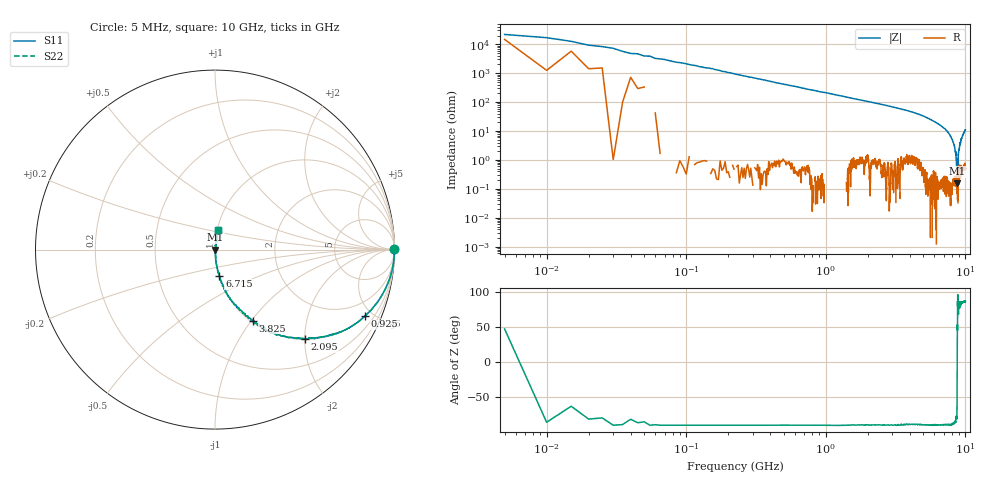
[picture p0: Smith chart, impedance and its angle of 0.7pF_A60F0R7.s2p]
! Amotech Co.,Ltd.
! http://www.amotech.co.kr/
! Part Number: A60F0R7
! These Parameters are Measured in Series Mode Connection
! Operation Temp=25[degC], DC Bias Voltage=0[V]
! Freq. Start=5[MHz] Stop=10[GHz], 2000[Steps]
! Date: Monday, July 20, 2020, 03:12:17
# GHZ S RI R 50.000000
!Freq.(Hz) S11(Real) S11(Imag) S21(Real) S21(Imag) S12(Real) S12(Imag) S22(Real) S22(Imag)
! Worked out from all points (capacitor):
!   2000 points, 5 MHz to 10 GHz, reference 50 ohm
!   read as one part in series: C = 763 fF near 55 MHz
!   lowest |Z| = 158 mohm at 8.72 GHz (marker M1)
!   series resonance near 8.732 GHz, so ESL is about 440 pH
!   S11 on the Smith chart (normalised r, x): 5 MHz: open; 925 MHz: 1.00, -4.51; 2.095 GHz: 1.01, -2.01; 3.825 GHz: 1.02, -1.02; 6.715 GHz: 1.00, -0.30; 10 GHz: 1.01, +0.22
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0.005  0.9969 0.00336  0.00309 -0.00336  0.00309 -0.00336  0.9969 0.00336
0.09  0.9981 -0.0431  0.00188 0.0431  0.00188 0.0431  0.9981 -0.0431
0.24  0.9871 -0.1127  0.0129 0.1127  0.0129 0.1127  0.9871 -0.1127
0.49  0.9464 -0.2241  0.0536 0.2241  0.0536 0.2241  0.9464 -0.2241
0.925  0.8355 -0.3706  0.1645 0.3706  0.1645 0.3706  0.8355 -0.3706
1.675  0.6107 -0.4846  0.3893 0.4846  0.3893 0.4846  0.6107 -0.4846
2.095  0.502 -0.497  0.498 0.497  0.498 0.497  0.502 -0.497
3.34  0.2652 -0.4395  0.7348 0.4395  0.7348 0.4395  0.2652 -0.4395
3.825  0.2106 -0.3959  0.7894 0.3959  0.7894 0.3959  0.2106 -0.3959
5.005  0.0985 -0.2934  0.9015 0.2934  0.9015 0.2934  0.0985 -0.2934
6.67  0.0246 -0.1502  0.9754 0.1502  0.9754 0.1502  0.0246 -0.1502
6.715  0.0241 -0.1466  0.9759 0.1466  0.9759 0.1466  0.0241 -0.1466
7.7  0.00689 -0.0771  0.9931 0.0771  0.9931 0.0771  0.00689 -0.0771
8.335  0.00288 -0.0305  0.9971 0.0305  0.9971 0.0305  0.00288 -0.0305
8.545  0.00242 -0.0148  0.9976 0.0148  0.9976 0.0148  0.00242 -0.0148
8.72  0.00128 -0.000914  0.9987 0.000914  0.9987 0.000914  0.00128 -0.000914
8.755  0.00418 0.00265  0.9958 -0.00265  0.9958 -0.00265  0.00418 0.00265
8.815  -0.000866 0.00785  1.001 -0.00785  1.001 -0.00785  -0.000866 0.00785
8.935  0.0066 0.0179  0.9934 -0.0179  0.9934 -0.0179  0.0066 0.0179
9.135  0.00698 0.034  0.993 -0.034  0.993 -0.034  0.00698 0.034
9.515  0.01 0.0656  0.99 -0.0656  0.99 -0.0656  0.01 0.0656
10  0.0167 0.1071  0.9833 -0.1071  0.9833 -0.1071  0.0167 0.1071
